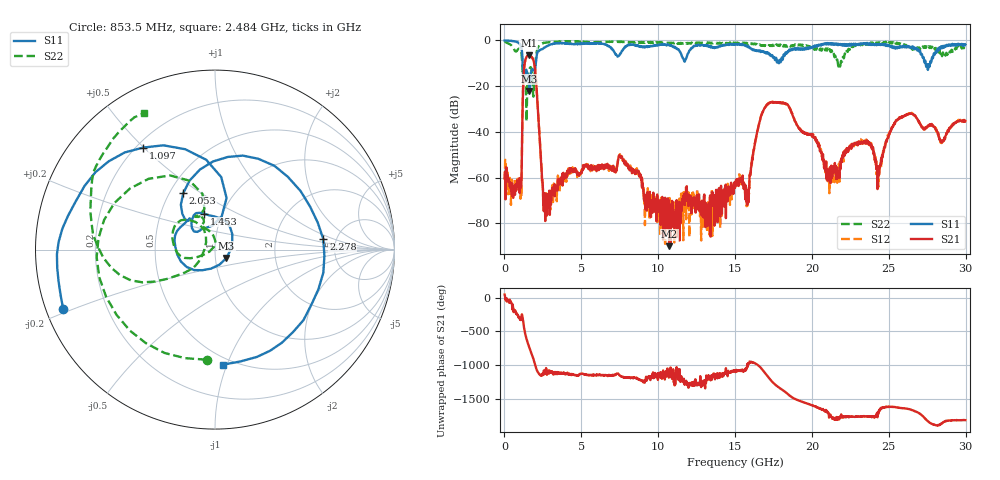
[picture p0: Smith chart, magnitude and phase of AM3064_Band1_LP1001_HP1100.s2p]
# Hz S DB R 50.0
!freq dBS11 angS11 dBS21 angS21 dBS12 angS12 dBS22 angS22
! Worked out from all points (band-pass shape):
!   1600 points, 10 MHz to 29.98 GHz, reference 50 ohm
!   highest |S21| = -6.53 dB at 1.584 GHz (marker M1); lowest = -90.0 dB at 10.71 GHz (marker M2)
!   |S21| within 3 dB of the highest: 1.329 GHz to 1.917 GHz (587.8 MHz wide, 36.2 % of centre)
!   lowest |S11| = -22.1 dB at 1.622 GHz (marker M3), VSWR 1.17, Z = 56.5 - j5.31 ohm
!   |S11| at or under -10 dB: 1.187 GHz to 2.035 GHz (848.4 MHz wide, 52.7 % of centre); 17.84888 GHz to 17.85512 GHz (6.245 MHz wide, 0.035 % of centre); 27.4 GHz to 27.68 GHz (282.8 MHz wide, 1.03 % of centre)
!   |S22| runs from -35.4 to -0.4 dB; largest |S21 - S12| = 0.0057
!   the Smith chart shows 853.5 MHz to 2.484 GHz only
!   S11 on the Smith chart (normalised r, x): 853.5 MHz: 0.05, -0.19; 1.097 GHz: 0.23, +0.50; 1.453 GHz: 0.82, +0.34; 2.053 GHz: 0.59, +0.42; 2.278 GHz: 3.94, +0.73; 2.484 GHz: 0.44, -0.97
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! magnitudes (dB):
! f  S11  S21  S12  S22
! 10 MHz  -0.1  -60.1  -60.2  -0.4
! 853.5 MHz  -0.8  -62.1  -60.5  -4.2
! 1.097 GHz  -3.2  -62.9  -68.3  -5.3
! 1.453 GHz  -13.6  -7.1  -7.0  -29.9
! 1.584 GHz  -19.6  -6.5  -6.5  -13.1
! 1.622 GHz  -22.1  -6.6  -6.5  -12.5
! 2.053 GHz  -8.8  -17.3  -17.3  -7.1
! 2.278 GHz  -4.3  -41.5  -41.7  -1.9
! 2.484 GHz  -3.8  -62.7  -62.5  -1.3
! 5.015 GHz  -1.4  -57.8  -57.9  -0.7
! 7.582 GHz  -5.5  -51.4  -50.9  -0.5
! 10 GHz  -2.0  -70.1  -74.5  -0.9
! 10.71 GHz  -2.0  -90.0  -80.3  -1.1
! 15 GHz  -1.8  -64.5  -62.9  -1.4
! 15.81 GHz  -2.9  -67.3  -72.3  -1.5
! 17.18 GHz  -5.5  -27.6  -27.5  -2.4
! 19.99 GHz  -3.4  -41.7  -41.6  -3.1
! 21.13 GHz  -1.2  -58.1  -66.8  -4.0
! 23.23 GHz  -1.8  -44.2  -42.9  -1.5
! 24.34 GHz  -2.0  -56.0  -57.3  -1.2
! 25 GHz  -2.1  -41.4  -40.9  -1.0
! 29.98 GHz  -1.8  -35.3  -35.4  -3.1
